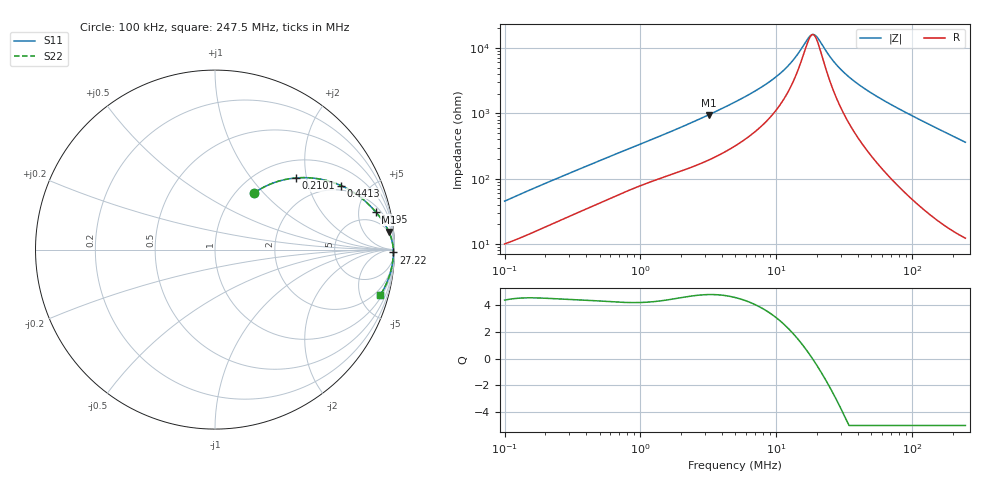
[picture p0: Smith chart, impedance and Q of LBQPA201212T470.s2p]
! LBQPA201212T470  S-PARAMETER MODEL  ( General Type )
! Model Generated by TAIYO YUDEN Corporation (http://www.ty-top.com)
! Version 1.0
! TAIYO YUDEN Control No. 191025NI43SB-FBB
! Copyright(c) 2019 TAIYO YUDEN CO.,LTD. All Rights Reserved.
! Product Description (link to TY-COMPAS)
! https://ds.yuden.co.jp/TYCOMPAS/or/detail?pn=LBQPA201212T470K&u=M
! Products Name : Inductors
! Characteristics :
!  Inductance : 47 uH , SRF(min) : 11 MHz , DC Resistance(max) : 7.54 Ohm
!  Rated Current : Saturation :120 mA , Temp Rise : 115 mA (20 degC)
!  Case Size : 2.0 x 1.25 / 0.079 x 0.049 [mm/inch] , Thickness : 1.25 / 0.049 [mm/inch]
!  (Conditions: Temperature = 25 degC , DC Bias Current/Voltage = 0A / 0V)
! External Node Assignments :
!  1  o---GGG---o  2
! GND o---------o GND
! Frequency Range : 0.1MHz  -  247.502633MHz  [ 402 STEP ]
# MHz S RI R 50
! Freq[MHz].  S11 Real  S11 Imag  S21 Real  S21 Imag  S12 Real  S12 Imag  S22 Real  S22 Imag
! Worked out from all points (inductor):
!   401 points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, 100 kHz to 247.5 MHz, reference 50 ohm
!   read as one part in series: L = 69.2 uH near 104 kHz
!   highest Q = 4.81 at 3.174 MHz (marker M1), where L = 46.4 uH
!   self-resonance near 18.42 MHz
!   S11 on the Smith chart (normalised r, x): 100 kHz: 1.20, +0.89; 210.1 kHz: 1.38, +1.74; 441.3 kHz: 1.76, +3.30; 1.195 MHz: 2.80, +7.67; 27.22 MHz: open; 247.5 MHz: 1.25, -7.22
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0.1  0.2182 0.3147  0.7818 -0.3147  0.7818 -0.3147  0.2182 0.3147
0.210083  0.4521 0.3993  0.5479 -0.3993  0.5479 -0.3993  0.4521 0.3993
0.37019  0.6487 0.3772  0.3513 -0.3772  0.3513 -0.3772  0.6487 0.3772
0.441347  0.7021 0.3569  0.2979 -0.3569  0.2979 -0.3569  0.7021 0.3569
0.705334  0.8152 0.2877  0.1848 -0.2877  0.1848 -0.2877  0.8152 0.2877
1.195258  0.8962 0.2094  0.1038 -0.2094  0.1038 -0.2094  0.8962 0.2094
1.370406  0.9115 0.1911  0.0885 -0.1911  0.0885 -0.1911  0.9115 0.1911
3.174381  0.969 0.0982  0.031 -0.0982  0.031 -0.0982  0.969 0.0982
4.974964  0.9818 0.0636  0.0182 -0.0636  0.0182 -0.0636  0.9818 0.0636
7.796878  0.9886 0.0376  0.0114 -0.0376  0.0114 -0.0376  0.9886 0.0376
10.65771  0.9914 0.0229  0.00864 -0.0229  0.00864 -0.0229  0.9914 0.0229
13.21257  0.9926 0.0138  0.00738 -0.0138  0.00738 -0.0138  0.9926 0.0138
17.03251  0.9936 0.00342  0.00641 -0.00342  0.00641 -0.00342  0.9936 0.00342
18.41681  0.9938 0.000261  0.00621 -0.000261  0.00621 -0.000261  0.9938 0.000261
19.1506  0.9939 -0.00132  0.00613 0.00132  0.00613 0.00132  0.9939 -0.00132
20.30646  0.994 -0.00371  0.00603 0.00371  0.00603 0.00371  0.994 -0.00371
27.22034  0.9942 -0.0161  0.00585 0.0161  0.00585 0.0161  0.9942 -0.0161
32.45257  0.994 -0.0242  0.00602 0.0242  0.00602 0.0242  0.994 -0.0242
39.45378  0.9935 -0.034  0.0065 0.034  0.0065 0.034  0.9935 -0.034
68.1772  0.9897 -0.0698  0.0103 0.0698  0.0103 0.0698  0.9897 -0.0698
132.4626  0.9733 -0.1411  0.0267 0.1411  0.0267 0.1411  0.9733 -0.1411
247.5026  0.9215 -0.2524  0.0785 0.2524  0.0785 0.2524  0.9215 -0.2524
